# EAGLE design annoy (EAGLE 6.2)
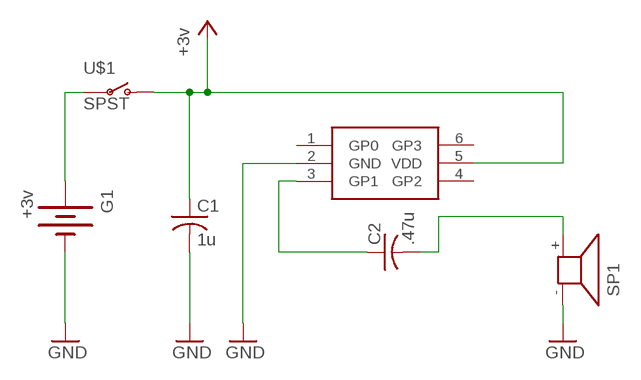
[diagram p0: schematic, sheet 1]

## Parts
C1  1u  C-USC1210  [C1210]
C2  .47u  C-USC1210  [C1210]
G1  +3v  BATTERY20PTH  [BATTCOM_20MM_PTH]
SP1  AL11P  [AL11P]
U$1  SPST  SWITCH-SPST-2TV  [SWITCH-SPST-VERTICAL]
U$2  PIC10  [PIC10]

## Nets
+3V3: C1.1 U$1.1(O) U$2.5(VDD) ; supply symbol labelled +3v
GND: C1.2 G1.2(-) SP1.- U$2.2(GND)
N$1: C2.1 U$2.3(GP1)
N$2: C2.2 SP1.+
N$4: G1.1(+) U$1.2(P)
Unconnected: U$2.1(GP0) U$2.4(GP2) U$2.6(GP3)

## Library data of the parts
C1 C2 = resistor:C-US: CAPACITOR, American symbol
G1 = SparkFun-Electromechanical:BATTERY: Battery Holders
SP1 = buzzer:AL11P: SPEAKER; OC_FARNELL: unknown; OC_NEWARK: unknown
U$1 = SparkFun-Electromechanical:SWITCH-SPST-2
U$2 = pyro_test:PIC10

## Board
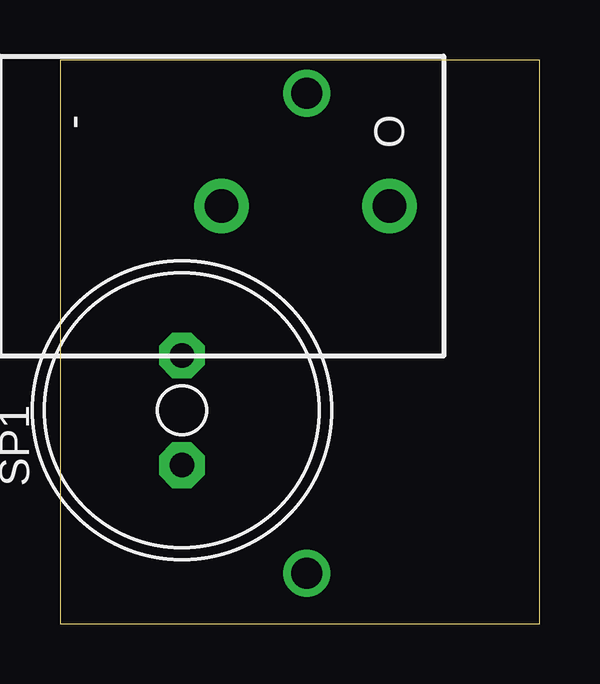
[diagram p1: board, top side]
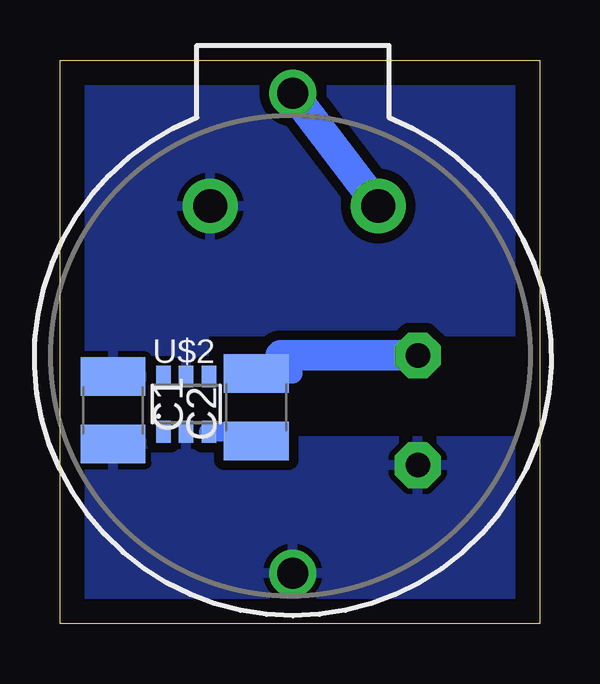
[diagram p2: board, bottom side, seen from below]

Size 19.99 x 23.48 mm. Coordinates in mm from the lower left corner, seen from the top.
Outline: 0,0 19.99,0 19.99,23.48 0,23.48 0,0
Copper layers (1*16): Top 0.035mm / dielectric 1.5mm / Bottom 0.035mm
Design rules: minimum track width 10mil, minimum drill 24mil, track to track 8mil, track to pad 8mil, pad to pad 8mil, via to via 8mil, smd to smd 8mil, copper to edge 40mil, drill to drill 8mil, minimum pad ring 10mil, minimum via ring 8mil, stop-mask expansion 4mil, vias tented up to drill 0mil, thermal gap 10mil

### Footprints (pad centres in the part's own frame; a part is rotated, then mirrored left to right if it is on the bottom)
C1210 = smd 1.6 x 2.7: 1 -1.4,0; 2 1.4,0
BATTCOM_20MM_PTH = drill 1.3: 1 20,0; 2 0,0
AL11P = drill 1.016 pad 1.905 octagon: + 2.286,0; - -2.286,0
SWITCH-SPST-VERTICAL = drill 1.4 pad 2.286: 1 0,7; 2 0,0
PIC10 = smd 0.6 x 0.9: 1 -0.95,-1.15; 2 0,-1.15; 3 0.95,-1.15; 4 0.95,1.15; 5 0,1.15; 6 -0.95,1.15

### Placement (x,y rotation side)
C1  17.78,8.89 270 bottom
C2  11.81,9.02 90 bottom
G1  10.29,2.1 90 bottom
SP1  5.08,8.89 90 top
U$1  6.73,17.4 270 top
U$2  14.73,9.14 0 bottom

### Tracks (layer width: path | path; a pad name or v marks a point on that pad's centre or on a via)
+3V3
  pour Bottom (isolate 0.406): 0,23.5 20.32,23.5 20.32,10.16 13.97,10.16 13.97,12.19 0,12.19
GND
  pour Bottom (isolate 0.406): 0,0 20.32,0 20.32,7.62 0,7.62
N$1
  Bottom 0.61: 11.81,7.87 C2.1
  Bottom 0.813: U$2.3 11.81,7.99 C2.1
N$2
  Bottom 0.813: 11.55,10.42 10.29,10.42 10.29,11.18
  Bottom 1.27: C2.2 11.55,10.42 | 10.79,11.18 10.29,11.18 SP1.+
N$4
  Bottom 1.27: G1.1 7.11,17.91 U$1.2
